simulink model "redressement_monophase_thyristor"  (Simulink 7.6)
settings: Solver=FixedStepDiscrete  StartTime=0.0  StopTime=0.05  RelTol=1e-3
InitFcn:
  | clc
  | clear all
  | close all
  | Ts=1e-5;
  | N=0.05;
StopFcn:
  | subplot 211
  | load iAK_vAK.mat
  | plot(x(1,:),x(2,:))
  | grid
  | title('Courant iAK - redressement monophasé à thyristor')
  | axis([0 N -1 11])
  | 
  | subplot 212
  | plot(x(1,:),x(3,:))
  | xlabel('temps')
  | title('Tension vAK - redressement monophasé à thyristor')
  | grid
  | axis([0 N -110 100])
  | 
  | figure
  | load Ug_vs.mat
  | subplot 211
  | plot(y(1,:),y(2,:))
  | title('Tension de sortie vs - redressement monophasé à thyristor')
  | axis([0 N -20 120])
  | grid
  | 
  | subplot 212
  | plot(y(1,:),y(3,:))
  | grid
  | axis([0 N -0.2 1.2])
  | title('Tension de commande de la gâchette - redressement monophasé à thyristor')
  | xlabel('temps')
undefined symbols (not defined in the file or in its folder): y
libraries: powerlib x8, powerlib_extras x1

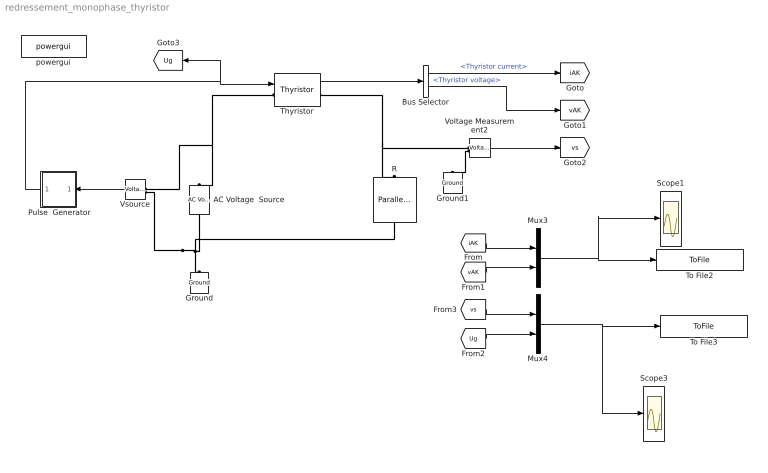
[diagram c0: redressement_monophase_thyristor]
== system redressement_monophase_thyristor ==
  " Pulse  Generator" : Subsystem
  AC Voltage  Source : powerlib/Electrical Sources/AC Voltage Source  DialogController=POWERSYS.PowerSysDialog  SystemSampleTime=-1  Amplitude=100  Phase=0  Frequency=60  SampleTime=Ts  Measurements=None
  Bus Selector : BusSelector  OutputSignals=Thyristor current,Thyristor voltage
  Ground : powerlib/Elements/Ground  DialogController=POWERSYS.PowerSysDialog  PhysicalDomain=powersysdomain  SubClassName=unknown  LeftPortType=p1  RightPortType=p1  LConnTagsString=a
  Ground1 : powerlib/Elements/Ground  DialogController=POWERSYS.PowerSysDialog  PhysicalDomain=powersysdomain  SubClassName=unknown  LeftPortType=p1  RightPortType=p1  LConnTagsString=a
  Mux3 : Mux  Inputs=2
  Mux4 : Mux  Inputs=2
  R : powerlib/Elements/Parallel RLC Branch  DialogController=POWERSYS.PowerSysDialog  PhysicalDomain=powersysdomain  SubClassName=unknown  LeftPortType=p1  RightPortType=p1  LConnTagsString=a  RConnTagsString=__new0  BranchType=R  Resistance=10  Inductance=1e-3  SetiL0=off  InitialCurrent=0  Capacitance=1e-6  Setx0=off  InitialVoltage=0  Measurements=None
  Scope1 : Scope
  Scope3 : Scope
  Thyristor : powerlib/Power Electronics/Thyristor  DialogController=POWERSYS.PowerSysDialog  SystemSampleTime=-1  Ron=0.001  Lon=0  Vf=0.8  IC=0  Rs=500  Cs=250e-9  Measurements=on
  To File2 : ToFile  Filename=iAK_vAK  MatrixName=x
  To File3 : ToFile  Filename=Ug_vs  MatrixName=y
  Voltage Measurement2 : powerlib/Measurements/Voltage Measurement  DialogController=POWERSYS.PowerSysDialog  SystemSampleTime=-1  PhasorSimulation=off  OutputType=Complex  PSBequivalent=0
  Vsource : powerlib/Measurements/Voltage Measurement  Tag=PoWeRsYsTeMmEaSuReMeNt  DialogController=POWERSYS.PowerSysDialog  SystemSampleTime=-1  PhasorSimulation=off  OutputType=Magnitude  PSBequivalent=0
  powergui : powerlib/powergui  SystemSampleTime=-1  SimulationMode=Discrete  SampleTime=Ts  frequency=60  SPID=off  DisableSnubberDevices=off  DisableRonSwitches=off  DisableVfSwitches=off  SwTol=0  Interpol=off  frequencyindice=0  echomessages=off  HookPort=off  DisplayEquations=off  FunctionMessages=off  EnableUseOfTLC=off  x0status=blocks  RestoreLinks=warning  ResistiveCurrentMeasurement=off  Frange=[0:2:500]  Ylog=off  Xlog=on  ShowGrid=off  save=off  variable=ZData  ZoomFFT=on  StartTime=0.0  cycles=1  DisplayStyle=1  fundamental=60  FreqAxis=off  MaxFrequency=1000  frequencyindicesteady=60  RmsSteady=1  display=off  Ts=0  methode=off
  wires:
  Thyristor/1 -> Bus Selector/1
  Bus Selector/1 -> [iAK]  "<Thyristor current>"
  Bus Selector/2 -> [vAK]  "<Thyristor voltage>"
  Voltage Measurement2/1 -> [vs]
  [iAK] -> Mux3/1
  [vAK] -> Mux3/2
  Mux3/1 -> To File2/1, Scope1/1
  Mux4/1 -> To File3/1, Scope3/1
  Vsource/1 -> " Pulse  Generator"/1(vs)
  " Pulse  Generator"/1(Pulses) -> Thyristor/1, [Ug]
  [Ug] -> Mux4/2
  [vs] -> Mux4/1
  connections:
  Vsource/LConn2 -- R/RConn1 -- AC Voltage  Source/LConn1 -- Ground/LConn1
  Thyristor/LConn1 -- AC Voltage  Source/RConn1 -- Vsource/LConn1
  Thyristor/RConn1 -- R/LConn1 -- Voltage Measurement2/LConn1
  Voltage Measurement2/LConn2 -- Ground1/LConn1

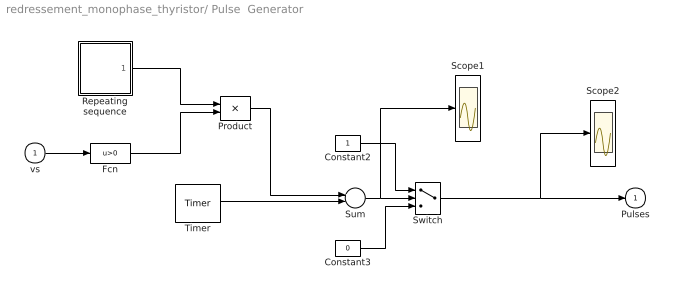
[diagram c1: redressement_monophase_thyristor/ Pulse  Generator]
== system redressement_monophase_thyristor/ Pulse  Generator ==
  vs : Inport
  Constant2 : Constant
  Constant3 : Constant  Value=0
  Fcn : Fcn  Expr=u>0
  Product : Product
  Repeating sequence : Subsystem  mask(Repeating table){t =[0 1/60 ],  y =[0 360 ]}
      mask prompts: t  "Time values:";  y  "Output values:"
      mask help: Repeating table. Enter values of time and output for first cycle.
      mask init:
      | period = max(t);
  Scope1 : Scope
  Scope2 : Scope
  Sum : Sum  Inputs=+-
  Switch : Switch  Threshold=0.5
  Timer : powerlib_extras/Control  Blocks/Timer  DialogController=POWERSYS.PowerSysDialog  SystemSampleTime=-1  t="[ 0  1/60 2/60 3/60 4/60 ]"  e="[20   50   80   110  140  ]"
  Pulses : Outport  InitialOutput=0
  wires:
  Timer/1 -> Sum/2
  Constant3/1 -> Switch/3
  Switch/1 -> Pulses/1, Scope2/1
  Sum/1 -> Switch/2, Scope1/1
  Constant2/1 -> Switch/1
  Repeating sequence/1(out_1) -> Product/1
  Fcn/1 -> Product/2
  vs/1 -> Fcn/1
  Product/1 -> Sum/1

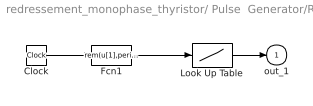
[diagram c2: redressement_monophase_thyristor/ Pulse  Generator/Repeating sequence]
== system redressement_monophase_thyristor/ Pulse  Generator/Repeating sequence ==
  Clock : Clock
  Fcn1 : Fcn  Expr=rem(u[1],period)
  Look Up Table : Lookup  InputValues=t  Table=y
  out_1 : Outport  InitialOutput=0
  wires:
  Fcn1/1 -> Look Up Table/1
  Clock/1 -> Fcn1/1
  Look Up Table/1 -> out_1/1
